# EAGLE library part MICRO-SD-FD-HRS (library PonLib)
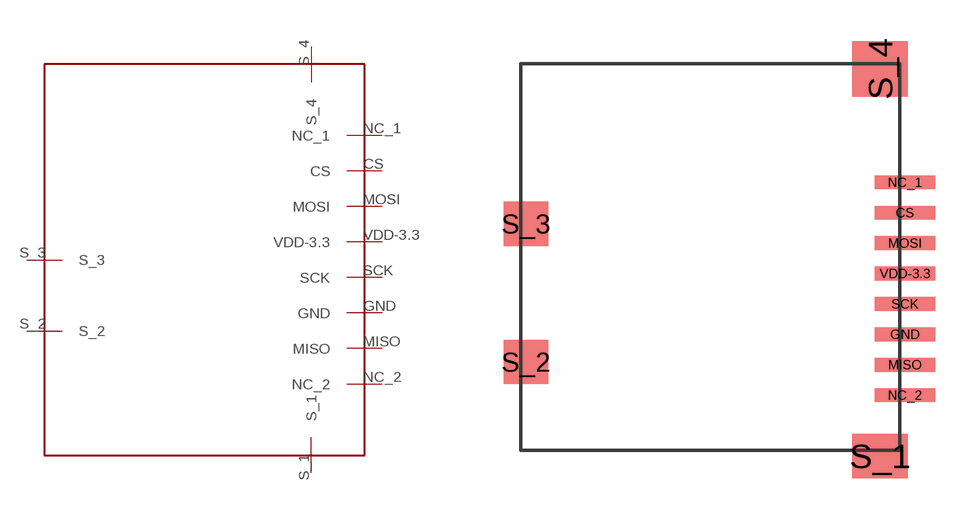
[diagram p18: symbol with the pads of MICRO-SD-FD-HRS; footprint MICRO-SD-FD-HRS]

Designator prefix -

## MICRO-SD-FD-HRS  [MICRO-SD-FD-HRS]
CS  CS
GND  GND
MISO  MISO
MOSI  MOSI
NC_1  NC_1
NC_2  NC_2
S_1  S_1
S_2  S_2
S_3  S_3
S_4  S_4
SCK  SCK
VDD-3.3  VDD-3.3

## Footprint MICRO-SD-FD-HRS (pad centres in mm)
smd 2.2 x 0.5: CS 6.9,1.6; GND 6.9,-2.8; MISO 6.9,-3.9; MOSI 6.9,0.5; NC_1 6.9,2.7; NC_2 6.9,-5; SCK 6.9,-1.7; VDD-3.3 6.9,-0.6
smd 2 x 1.6: S_1 6,-7.2
smd 1.6 x 1.6: S_2 -6.8,-3.8; S_3 -6.8,1.2
smd 2 x 2: S_4 6,6.8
